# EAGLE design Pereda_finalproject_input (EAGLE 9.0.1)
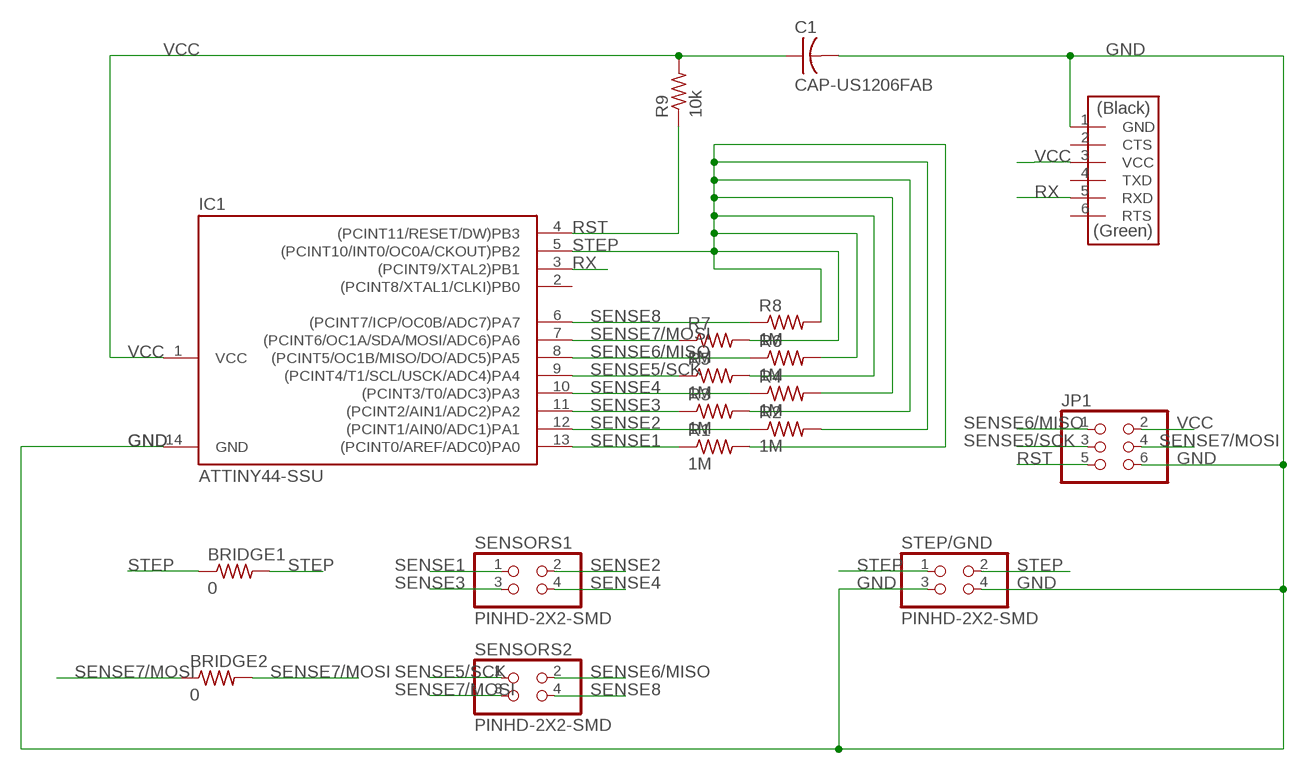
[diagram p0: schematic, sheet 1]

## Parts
BRIDGE1  0  RES-US1206FAB  [R1206FAB]
BRIDGE2  0  RES-US1206FAB  [R1206FAB]
C1  CAP-US1206FAB  [C1206FAB]
IC1  ATTINY44-SSU  [SOIC14]
JP1  PINHD-2X3-SMD  [2X03SMD]
R1  1M  RES-US1206FAB  [R1206FAB]
R2  1M  RES-US1206FAB  [R1206FAB]
R3  1M  RES-US1206FAB  [R1206FAB]
R4  1M  RES-US1206FAB  [R1206FAB]
R5  1M  RES-US1206FAB  [R1206FAB]
R6  1M  RES-US1206FAB  [R1206FAB]
R7  1M  RES-US1206FAB  [R1206FAB]
R8  1M  RES-US1206FAB  [R1206FAB]
R9  10k  RES-US1206FAB  [R1206FAB]
SENSORS1  PINHD-2X2-SMD  [2X02SMD]
SENSORS2  PINHD-2X2-SMD  [2X02SMD]
STEP/GND  PINHD-2X2-SMD  [2X02SMD]
U$4  FTDI-SMD-HEADER  [1X06SMD]

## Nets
GND: C1.2 IC1.14(GND) JP1.6 STEP/GND.3 STEP/GND.4 U$4.1(GND)
RST: IC1.4((PCINT11/RESET/DW)PB3) JP1.5 R9.1
RX: IC1.3((PCINT9/XTAL2)PB1) U$4.5(RXD)
SENSE1: IC1.13((PCINT0/AREF/ADC0)PA0) R1.1 SENSORS1.1
SENSE2: IC1.12((PCINT1/AIN0/ADC1)PA1) R2.1 SENSORS1.2
SENSE3: IC1.11((PCINT2/AIN1/ADC2)PA2) R3.1 SENSORS1.3
SENSE4: IC1.10((PCINT3/T0/ADC3)PA3) R4.1 SENSORS1.4
SENSE5/SCK: IC1.9((PCINT4/T1/SCL/USCK/ADC4)PA4) JP1.3 R5.1 SENSORS2.1
SENSE6/MISO: IC1.8((PCINT5/OC1B/MISO/DO/ADC5)PA5) JP1.1 R6.1 SENSORS2.2
SENSE7/MOSI: BRIDGE2.1 BRIDGE2.2 IC1.7((PCINT6/OC1A/SDA/MOSI/ADC6)PA6) JP1.4 R7.1 SENSORS2.3
SENSE8: IC1.6((PCINT7/ICP/OC0B/ADC7)PA7) R8.1 SENSORS2.4
STEP: BRIDGE1.1 BRIDGE1.2 IC1.5((PCINT10/INT0/OC0A/CKOUT)PB2) R1.2 R2.2 R3.2 R4.2 R5.2 R6.2 R7.2 R8.2 STEP/GND.1 STEP/GND.2
VCC: C1.1 IC1.1(VCC) JP1.2 R9.2 U$4.3(VCC)
Unconnected: IC1.2((PCINT8/XTAL1/CLKI)PB0) U$4.2(CTS) U$4.4(TXD) U$4.6(RTS)

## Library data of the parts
BRIDGE1 BRIDGE2 R1-R9 = fablibrary:RES-US: Resistor (US Symbol)
C1 = fablibrary:CAP-US
IC1 = fablibrary:ATTINY44
JP1 = fablibrary:PINHD-2X3-SMD: PIN HEADER
SENSORS1 SENSORS2 STEP/GND = fablibrary:PINHD-2X2-SMD
U$4 = fablibrary:FTDI-SMD-HEADER

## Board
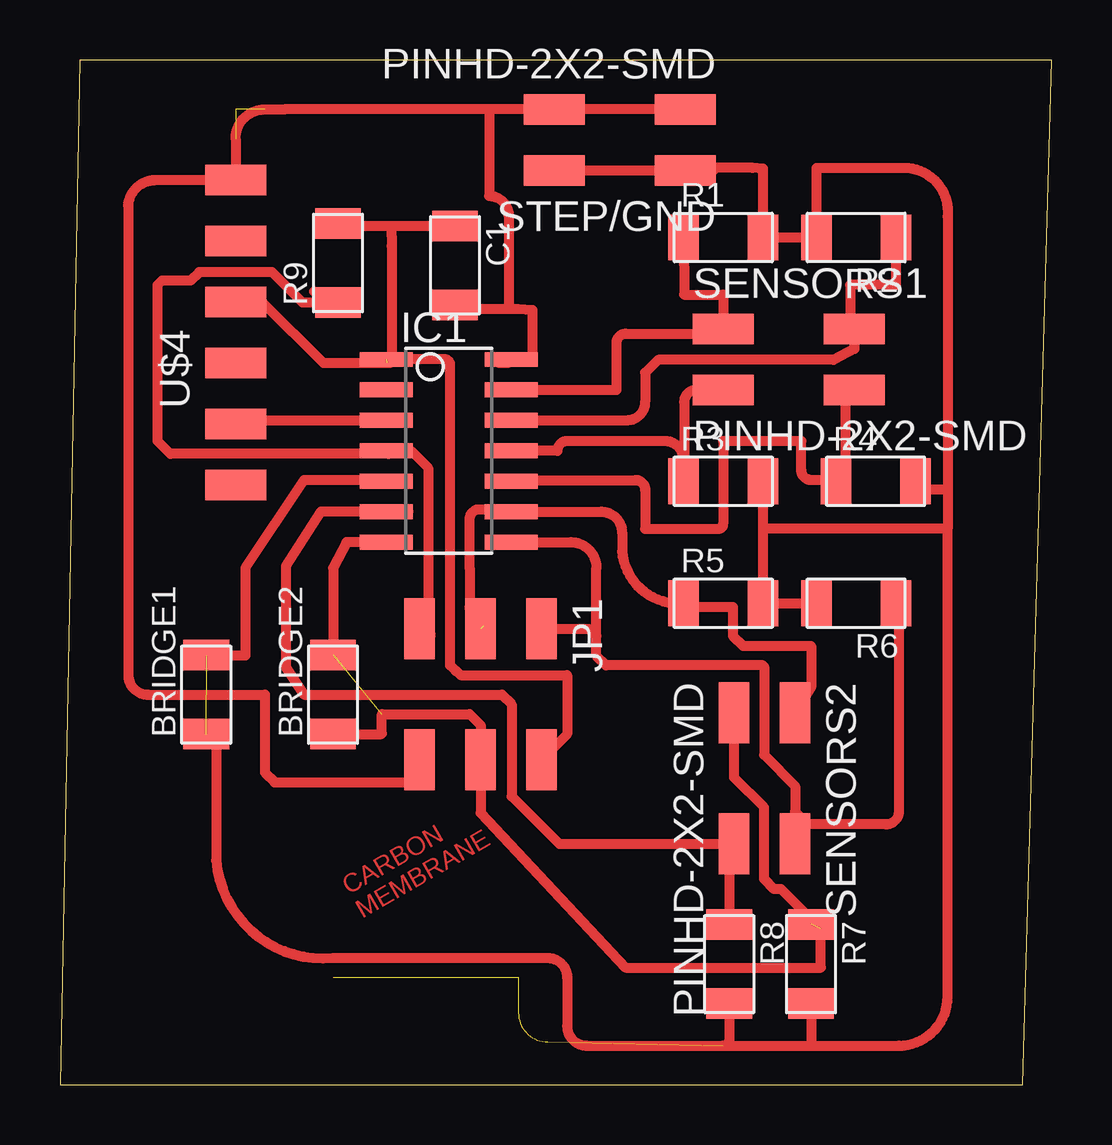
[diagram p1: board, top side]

Size 41.33 x 42.7 mm. Coordinates in mm from the lower left corner, seen from the top.
Outline: 0,0 40.11,0 41.33,42.7 0.81,42.7 0,0
Copper layers (1*16): Top 0.035mm / dielectric 1.5mm / Bottom 0.035mm
Design rules "default *": minimum track width 16mil, minimum drill 0.35mm, track to track 16mil, track to pad 16mil, pad to pad 16mil, via to via 16mil, smd to smd 16mil, copper to edge 40mil, drill to drill 6mil, minimum pad ring 10mil, minimum via ring 8mil, stop-mask expansion 4mil, vias tented up to drill 0mil, thermal gap 10mil

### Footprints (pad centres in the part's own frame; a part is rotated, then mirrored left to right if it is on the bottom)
R1206FAB = smd 1.27 x 1.905: 1 -1.651,0; 2 1.651,0
C1206FAB = smd 1.27 x 1.905: 1 -1.651,0; 2 1.651,0
SOIC14 = smd 0.61 x 2.21: 1 -3.81,-2.603; 2 -2.54,-2.603; 3 -1.27,-2.603; 4 0,-2.603; 5 1.27,-2.603; 6 2.54,-2.603; 7 3.81,-2.603; 8 3.81,2.603; 9 2.54,2.603; 10 1.27,2.603; 11 0,2.603; 12 -1.27,2.603; 13 -2.54,2.603; 14 -3.81,2.603
2X03SMD = smd 2.54 x 1.27: 1 -2.54,2.54; 2 2.92,2.54; 3 -2.54,0; 4 2.92,0; 5 -2.54,-2.54; 6 2.92,-2.54
2X02SMD = smd 2.54 x 1.27: 1 -2.54,1.27; 2 2.92,1.27; 3 -2.54,-1.27; 4 2.92,-1.27
1X06SMD = smd 2.54 x 1.27: 1 0,6.35; 2 0,3.81; 3 0,1.27; 4 0,-1.27; 5 0,-3.81; 6 0,-6.35

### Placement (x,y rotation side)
BRIDGE1  6.1,16.26 90 top
BRIDGE2  11.38,16.26 90 top
C1  16.46,34.14 270 top
IC1  16.21,26.42 270 top
JP1  17.53,16.46 270 top
R1  27.64,35.31 0 top
R2  33.17,35.31 180 top
R3  27.64,25.15 0 top
R4  33.99,25.15 0 top
R5  27.64,20.07 0 top
R6  33.17,20.07 180 top
R7  31.29,5.03 270 top
R8  27.89,5.03 270 top
R9  11.58,34.24 90 top
SENSORS1  30.18,30.23 0 top
SENSORS2  29.36,12.95 270 top
STEP/GND  23.52,39.37 180 top
U$4  7.32,31.34 0 top

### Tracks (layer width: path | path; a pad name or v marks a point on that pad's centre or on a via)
GND  (2 unrouted)
  Top 0.406: 18.29,30.07 18.66,30.07 IC1.14 19.69,30.23 19.69,32.28 19.09,32.33 18.69,32.33 | C1.2 16.87,32.33 18.69,32.33 | STEP/GND.3 STEP/GND.4 17.88,40.64 | 17.88,40.64 9.35,40.64 8.53,40.64 arc90 7.32,39.42 U$4.1 3.96,37.69 arc90 2.85,36.58 2.85,17.07 arc90 3.66,16.26 8.53,16.26 8.53,13 8.94,12.6 15.04,12.6 15.04,13 14.99,13.06 JP1.6 | 17.88,40.64 17.88,37.03 arc-90 18.69,36.22 18.69,32.33
RST
  Top 0.406: 10.59,33.05 R9.1 10.11,32.59 8.84,33.86 5.79,33.86 5.44,33.5 4.24,33.5 4.06,33.33 4.06,26.82 4.6,26.29 13.69,26.29 13.82,26.42 IC1.4 | 13.01,26.42 IC1.4 | 15.44,18.69 arc90 15.14,19 JP1.5 15.34,19.36 15.34,25.7 14.63,26.42 IC1.4
RX
  Top 0.406: U$4.5 7.47,27.69 IC1.3
SENSE1
  Top 0.406: 26.37,35.31 R1.1 26.01,32.92 27.64,32.92 SENSORS1.1 arc-90 27.43,31.29 23.57,31.29 arc90 23.19,30.91 23.19,28.96 IC1.13
SENSE2
  Top 0.406: 32.72,31.5 SENSORS1.2 | IC1.12 23.62,27.69 arc90 24.38,28.45 24.38,29.67 24.92,30.2 32.23,30.2 33.1,30.66 SENSORS1.2 | 32.89,31.7 arc-90 SENSORS1.2 | 32.11,31.7 arc90 32.31,31.5 SENSORS1.2 | R2.1 34.82,33.33 32.92,33.33 32.92,31.5 SENSORS1.2
SENSE3
  Top 0.406: 26.37,25.15 R3.1 | 25.73,25.15 R3.1 | SENSORS1.3 26.52,28.96 arc90 26.01,28.45 26.01,25.17 arc-90 R3.1 | R3.1 25.98,26.04 arc90 25.2,26.82 21.13,26.82 arc90 20.73,26.42 IC1.11
SENSE4
  Top 0.406: R4.1 32.72,25.15 32.72,28.96 SENSORS1.4 | 32.08,25.15 R4.1 | R4.1 arc90 32.28,25.2 31.29,25.2 arc-90 30.89,25.6 30.89,26.82 27.64,26.82 27.64,23.37 arc-90 27.43,23.16 24.38,23.16 24.38,24.79 arc90 23.98,25.2 18.86,25.2 arc90 IC1.10
SENSE5/SCK  (1 unrouted)
  Top 0.406: 17.63,19.1 17.88,19.1 arc-90 17.07,19.91 17.07,21.54 17.07,21.95 17.07,23.57 arc-90 17.48,23.98 18.29,23.98 arc90 18.39,23.88 IC1.9 22.56,23.88 arc-90 23.42,23.01 23.42,22.23 arc90 R5.1 arc90 26.14,19.91 28.04,19.91 28.04,18.69 28.45,18.29 31.29,18.29 31.29,16.56 SENSORS2.1
SENSE6/MISO
  Top 0.406: IC1.8 21.29,22.61 arc-90 22.35,21.54 22.35,18.69 | 22.35,18.69 22.35,17.88 22.76,17.48 29.29,17.48 29.34,17.42 29.34,13.74 30.63,12.45 30.63,11.38 | R6.1 arc-90 34.95,19.94 34.95,11.38 arc-90 34.42,10.85 31.17,10.85 30.63,11.38 | 30.48,11 arc90 SENSORS2.2 30.63,11.38 | JP1.1 22.05,19 22.35,18.69
SENSE7/MOSI  (2 unrouted)
  Top 0.406: IC1.7 11.94,22.61 11.38,21.54 BRIDGE2.2 | JP1.4 17.35,13.54 | JP1.4 17.53,11.33 23.57,4.88 31.7,4.88 31.7,6.5 30.05,8.15 29.75,8.15 29.34,8.56 29.34,11.56 28.09,12.8 SENSORS2.3 | BRIDGE2.1 13.39,14.61 13.41,14.63 13.41,15.44 17.07,15.44 17.53,14.99 JP1.4
SENSE8
  Top 0.406: 13.5,23.98 arc-90 IC1.6 | IC1.6 14.53,23.88 | R8.1 27.89,10.64 arc-90 SENSORS2.4 20.8,10.03 18.82,12.02 18.82,15.85 18.42,16.26 10.17,16.26 9.41,17.43 9.41,21.6 10.87,23.88 IC1.6
STEP  (5 unrouted)
  Top 0.406: 35.89,25.15 R4.2 | 29.54,25.15 R3.2 29.29,23.16 | 35.26,25.15 R4.2 | 28.91,35.31 R1.2 | 35.81,25.15 R4.2 | R4.2 arc-90 35.76,25.02 35.76,24.79 36.98,24.79 | R1.2 29.29,38.18 28.85,38.2 27.23,38.2 27.23,38.1 STEP/GND.1 | 36.98,24.79 36.98,23.16 | STEP/GND.2 STEP/GND.1 | STEP/GND.1 26.06,38.2 | R1.2 R2.2 31.52,38.2 35.36,38.2 arc-90 36.98,36.17 36.98,24.79 | 29.29,23.16 R5.2 R6.2 | 36.98,23.16 29.29,23.16 | 13.55,25.2 arc-90 IC1.5 13.55,25.2 | 27.64,1.63 31.29,1.63 | 31.29,1.63 34.95,1.63 arc90 36.98,3.66 36.98,23.16 | R7.2 31.29,1.63 | R8.2 27.89,1.88 arc-90 27.64,1.63 | 13.55,25.2 10.16,25.2 7.72,21.54 7.72,17.88 6.12,17.88 BRIDGE1.2 | BRIDGE1.1 arc-90 6.5,14.2 6.5,9.35 arc90 11.38,5.28 20.32,5.28 arc-90 21.13,4.47 21.13,2.44 arc90 21.95,1.63 27.64,1.63
VCC  (1 unrouted)
  Top 0.406: 12.4,35.79 R9.2 arc90 11.68,35.79 13.82,35.79 | U$4.3 8.43,32.61 10.97,30.07 13.61,30.07 13.82,30.28 13.82,34.95 13.82,35.38 13.82,35.79 | IC1.1 arc90 13.75,30.07 arc-90 IC1.1 | IC1.1 16.1,30.23 16.26,30.07 16.26,17.48 16.48,17.25 16.51,17.25 16.69,17.07 21.13,17.07 21.13,14.61 JP1.2 | 13.82,35.79 C1.1

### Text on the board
Top: CARBON / MEMBRANE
